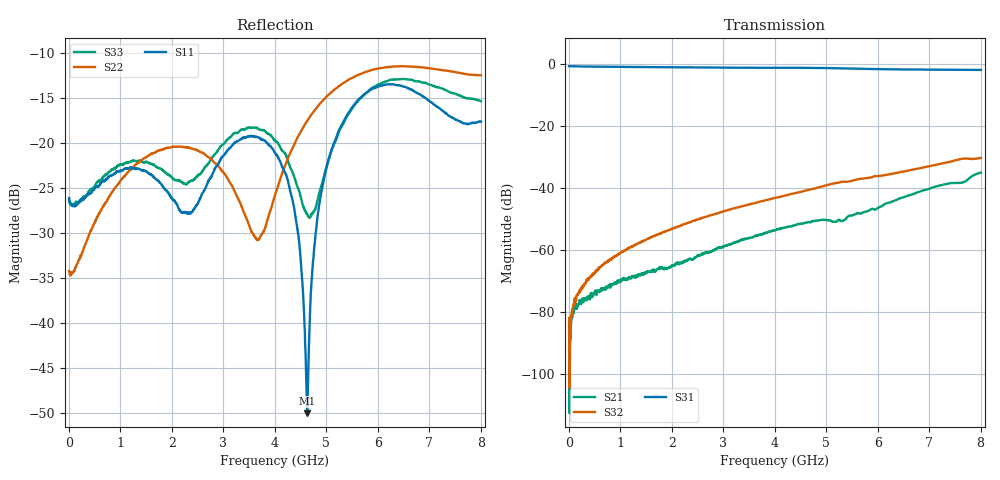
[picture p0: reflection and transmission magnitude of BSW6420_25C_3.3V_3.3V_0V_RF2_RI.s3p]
! Product: BSW6420
! Temp: 25C
! VDD: 3.300
! Control_Hi: 3.300
! Control_Lo: 0.000
! Logic State: RF2
! Port 1: RFC
! Port 2: RF1
! Port 3: RF2
! V1 = 0.00
! V2 = 0.00
! V3 = 0.00
! V4 = 0.00
# Hz S  RI  R 50
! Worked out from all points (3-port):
!   1601 points, 5 MHz to 8.005 GHz, reference 50 ohm
!   strongest paths, dB at 5 MHz, 2.005 GHz, 4.005 GHz, 6.005 GHz, 8.005 GHz:
!     S31: -0.6, -1.0, -1.1, -1.6, -1.8
!     S32: -82.0, -53.1, -43.2, -36.2, -30.2
!     S21: -84.2, -65.1, -53.6, -46.5, -35.0
!   lowest |S11| = -50.0 dB at 4.63 GHz (marker M1), VSWR 1.01, Z = 50.1 + j0.305 ohm
!   |S11| at or under -10 dB: start of sweep to end of sweep
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5000000  0.0492 -0.0037  3.71e-05 -7.32e-05  0.9329 -0.0116
         4.14e-05 -4.56e-05  0.0194 -0.00165  4.54e-05 -5.73e-05
         0.9331 -0.0116  4.52e-05 -6.51e-05  0.0485 -0.00352
8.8e8  -0.0484 -0.0468  0.000229 -0.000206  0.0177 -0.9113
       0.000205 -0.000187  -0.0428 -0.035  0.000731 0.00026
       0.0173 -0.9113  0.000745 0.000235  -0.0495 -0.0515
1.76e9  -0.0456 0.0395  -0.000462 -0.00021  -0.8968 -0.0481
        -0.000473 -0.000217  -0.0703 0.0575  0.00127 -0.00131
        -0.8972 -0.048  0.00127 -0.0013  -0.0588 0.0419
2.775e9  -0.0504 0.0411  0.000464 0.000833  0.1303 0.8776
         0.000461 0.000818  0.0448 0.0669  -0.0024 -0.00278
         0.1306 0.8777  -0.00239 -0.00277  -0.0408 0.0706
4.005e9  0.0571 0.0663  -0.000211 -0.00206  0.6614 -0.579
         -0.000191 -0.00207  -0.0474 -0.0196  -0.00333 0.00607
         0.6616 -0.5795  -0.00334 0.00609  0.0997 0.0225
4.63e9  0.000837 0.00304  -0.0027 -0.000664  -0.2164 -0.8501
        -0.00269 -0.000656  -0.095 0.0917  0.00442 0.00808
        -0.2167 -0.8502  0.00441 0.00805  -0.00981 -0.039
5.065e9  -0.05 0.068  -0.0024 0.00175  -0.74 -0.4536
         -0.00242 0.00178  -0.0365 0.1829  0.0107 0.00387
         -0.7401 -0.4534  0.0107 0.00389  -0.0585 0.0598
6.26e9  0.206 0.0461  0.00423 0.00414  -0.0214 0.8296
        0.00424 0.00412  0.262 0.0308  -0.00202 -0.0167
        -0.021 0.8296  -0.00206 -0.0168  0.2233 0.00739
7.145e9  -0.00763 -0.1587  0.00676 -0.00827  0.819 0.0324
         0.00676 -0.00828  0.0687 -0.246  -0.0237 0.00117
         0.819 0.0319  -0.0237 0.00118  0.0678 -0.1919
8.005e9  -0.0996 0.0849  -0.0132 -0.0118  0.0583 -0.809
         -0.0132 -0.0118  -0.2317 -0.05  0.00195 0.0308
         0.0581 -0.809  0.00205 0.0307  -0.1108 -0.1289
